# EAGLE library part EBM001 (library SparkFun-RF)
Bluetooth module
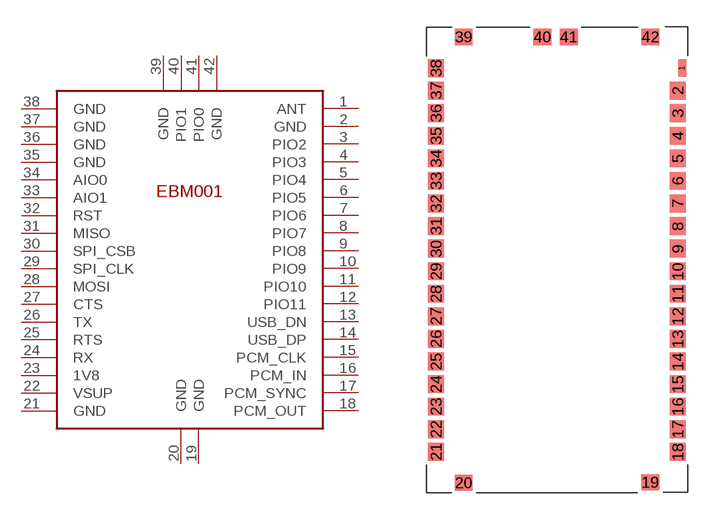
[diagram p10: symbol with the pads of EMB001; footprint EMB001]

Designator prefix -

## EBM001  [EMB001]
1  ANT
2  GND
3  PIO2
4  PIO3
5  PIO4
6  PIO5
7  PIO6
8  PIO7
9  PIO8
10  PIO9
11  PIO10
12  PIO11
13  USB_DN
14  USB_DP
15  PCM_CLK
16  PCM_IN
17  PCM_SYNC
18  PCM_OUT
19  GND
20  GND
21  GND
22  VSUP
23  1V8
24  RX
25  RTS
26  TX
27  CTS
28  MOSI
29  SPI_CLK
30  SPI_CSB
31  MISO
32  RST
33  AIO1
34  AIO0
35  GND
36  GND
37  GND
38  GND
39  GND
40  PIO1
41  PIO0
42  GND

## Footprint EMB001 (pad centres in mm)
smd 0.45 x 1: 1 13.83,0.01
smd 0.9 x 1: 2 13.6,-1.27; 3 13.6,-2.54; 4 13.6,-3.81; 5 13.6,-5.08; 6 13.6,-6.35; 7 13.6,-7.62; 8 13.6,-8.89; 9 13.6,-10.16; 10 13.6,-11.43; 11 13.6,-12.7; 12 13.6,-13.97; 13 13.6,-15.24; 14 13.6,-16.51; 15 13.6,-17.78; 16 13.6,-19.05; 17 13.6,-20.32; 18 13.6,-21.59; 21 0,-21.59; 22 0,-20.32; 23 0,-19.05; 24 0,-17.78; 25 0,-16.51; 26 0,-15.24; 27 0,-13.97; 28 0,-12.7; 29 0,-11.43; 30 0,-10.16; 31 0,-8.89; 32 0,-7.62; 33 0,-6.35; 34 0,-5.08; 35 0,-3.81; 36 0,-2.54; 37 0,-1.27; 38 0,0
smd 1 x 0.9: 19 12.05,-23.31; 20 1.55,-23.34; 39 1.55,1.75; 40 5.98,1.75; 41 7.46,1.75; 42 12.05,1.75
